PROGRAM PRG_METHOD
VAR
	(* Declarations for UA_Connect *)	
	fbUA_Connect: UA_Connect;
	SessionConnectInfo: ST_UASessionConnectInfo;
	nConnectionHdl: DWORD;
	
	(* Declarations for UA_GetNamespaceIndex *)
	fbUA_GetNamespaceIndex: UA_GetNamespaceIndex;
	nNamespaceIndex: UINT;
	
	(* Declarations for UA_MethodGetHandle *)
	fbUA_MethodGetHandle: UA_MethodGetHandle;
	ObjectNodeID: ST_UANodeID;
	MethodNodeID: ST_UANodeID;
	nMethodHdl: DWORD;
	
	(* Declarations for UA_MethodCall *)
	fbUA_MethodCall: UA_MethodCall;
	sObjectNodeIdIdentifier	: STRING(MAX_STRING_LENGTH) := 'MAIN.fbMathematics'; // change to object node identifier (UAObject above method)
	sMethodNodeIdIdentifier : STRING(MAX_STRING_LENGTH) := 'MAIN.fbMathematics#M_Mul'; // change to method node identifier (UAMethod to call)
	nAdrWriteData: PVOID;
	numberIn1: INT := 42; // change according to input value and data type
	numberIn2: INT := 42; // change according to input value and data type
	numberOutPro: DINT; // result (output parameter of M_Mul())
	cbWriteData: UDINT; // calculated automatically by M_Init()
	InputArguments: ARRAY[1..2] OF ST_UAMethodArgInfo; // change according to input parameters - M_Mul has 2 input parameters 
	stOutputArgInfo: ARRAY[1..1] OF ST_UAMethodArgInfo; // change according to output parameters - M_Mul has 1 output parameters
	stOutputArgInfoAndData: ST_OutputArgInfoAndData;
	nInputData: ARRAY[1..4] OF BYTE; // numberIn1(INT16)(2) + numberIn2(INT16)(2)
	nOffset: UDINT; // calculated by M_Init()
	nArg: INT; // used by M_Init()
	
	(* Declarations for UA_MethodReleaseHandle *)
	fbUA_MethodReleaseHandle: UA_MethodReleaseHandle;

	(* Declarations for UA_Disconnect *)
	fbUA_Disconnect: UA_Disconnect;
			
	(* Other Declarations *)
	bTest: BOOL := TRUE;
	bDone: BOOL;
	bBusy: BOOL;
	bError: BOOL;
	nErrorID: DWORD;
	iState: INT;
	RTrig: R_TRIG;
	bInputDataError: BOOL;
END_VAR
VAR CONSTANT
	nInputArgSize: INT := 4; // numberIn1(INT16)(2) + numberIn2(INT16)(2)
	nNumberOfInputArguments: DINT := 2; // change to number of input parameters - M_Mul has 2 input parameters
	nNumberOfOutputArguments: DINT := 1; // change to number of output parameters - M_Mul has 1 output parameters
END_VAR

CASE iState OF

0:	(* idle *)
	IF bTest THEN
		bTest		:= FALSE;
		bError		:= FALSE;
		nErrorID	:= 0;

		SessionConnectInfo.tConnectTimeout 		:= T#1M;
		SessionConnectInfo.tSessionTimeout 		:= T#1M;
		SessionConnectInfo.sApplicationName		:= '';
		SessionConnectInfo.eSecurityMode 		:= eUASecurityMsgMode_None;
		SessionConnectInfo.eSecurityPolicyUri 	:= eUASecurityPolicy_None;
		SessionConnectInfo.eTransportProfileUri := eUATransportProfileUri_UATcp;

		iState	:= iState + 1;
	END_IF

	
1:	(* open UA session *)
	fbUA_Connect(
		Execute				:= TRUE,
		ServerURL			:= sOpcUaServerUrl,
		SessionConnectInfo	:= SessionConnectInfo,
		Timeout				:= T#2M,
		ConnectionHdl		=> nConnectionHdl
	);

	IF NOT fbUA_Connect.Busy THEN
		fbUA_Connect(Execute := FALSE);

		IF NOT fbUA_Connect.Error THEN
			(* connected *)
			iState := iState + 1;
		ELSE
			bError			:= TRUE;
			nErrorID		:= fbUA_Connect.ErrorID;
			nConnectionHdl	:= 0;
			iState 			:= 0; (* idle *)
		END_IF
	END_IF


2:	(* GetNS Index *)
	fbUA_GetNamespaceIndex(
		Execute			:= TRUE,
		ConnectionHdl	:= nConnectionHdl,
		NamespaceUri	:= sNamespaceUri,
		NamespaceIndex	=> nNamespaceIndex
	);

	IF NOT fbUA_GetNamespaceIndex.Busy THEN
		fbUA_GetNamespaceIndex(Execute := FALSE);

		IF NOT fbUA_GetNamespaceIndex.Error THEN
			(* namespace index read successfully *)
			iState 		:= iState + 1;
		ELSE
			bError		:= TRUE;
			nErrorID	:= fbUA_GetNamespaceIndex.ErrorID;
			iState 		:= 7; (* disconnect *)
		END_IF
	END_IF

	
3:	(* Get Method Handle *)
	ObjectNodeID.eIdentifierType := eUAIdentifierType_String;
	ObjectNodeID.nNamespaceIndex := nNamespaceIndex;
	ObjectNodeID.sIdentifier	 := sObjectNodeIdIdentifier;

	MethodNodeID.eIdentifierType := eUAIdentifierType_String;
	MethodNodeID.nNamespaceIndex := nNamespaceIndex;
	MethodNodeID.sIdentifier	 := sMethodNodeIdIdentifier;

	M_Init();
	IF bInputDataError = FALSE THEN
		iState 	:= iState + 1;
	ELSE
		bBusy		:= FALSE;  
		bError 		:= TRUE;
		nErrorID 	:= 16#70A; //out of memory
	END_IF

	
4:	(* Method Get Handle *)
	fbUA_MethodGetHandle(
			Execute			:= TRUE,
			ConnectionHdl	:= nConnectionHdl,
			ObjectNodeID	:= ObjectNodeID,
			MethodNodeID 	:= MethodNodeID,
			MethodHdl		=> nMethodHdl
		);
	IF NOT fbUA_MethodGetHandle.Busy THEN
		fbUA_MethodGetHandle(Execute := FALSE);

		IF NOT fbUA_MethodGetHandle.Error THEN
			(*  *)
			iState := iState + 1; (* Call Method *)
		ELSE
			bError		:= TRUE;
			nErrorID	:= fbUA_MethodGetHandle.ErrorID;
			iState	 	:= 6; (* Release method Handle *)
		END_IF
	END_IF


5:	(* Method Call *)
	stOutputArgInfo[1].nLenData := SIZEOF(stOutputArgInfoAndData.pro);
	fbUA_MethodCall(
		Execute					:= TRUE,
		ConnectionHdl			:= nConnectionHdl,
		MethodHdl				:= nMethodHdl,
		nNumberOfInputArguments := nNumberOfInputArguments,	
		pInputArgInfo			:= ADR(InputArguments),
		cbInputArgInfo			:= SIZEOF(InputArguments),
		pInputArgData			:= ADR(nInputData),
		cbInputArgData			:= cbWriteData,
		pInputWriteData			:= 0,
		cbInputWriteData		:= 0,
		nNumberOfOutputArguments:= nNumberOfOutputArguments,
		pOutputArgInfo			:= ADR(stOutputArgInfo),
		cbOutputArgInfo			:= SIZEOF(stOutputArgInfo),
		pOutputArgInfoAndData	:= ADR(stOutputArgInfoAndData),
		cbOutputArgInfoAndData	:= SIZEOF(stOutputArgInfoAndData),		
	);
	IF NOT fbUA_MethodCall.Busy THEN
		fbUA_MethodCall(Execute := FALSE);
		IF NOT fbUA_MethodCall.Error THEN
			(* clear data and restart *)
			iState := iState + 1; (* Release handle *)
			numberOutPro := stOutputArgInfoAndData.pro;
		ELSE
			bError		:= TRUE;
			nErrorID	:= fbUA_MethodCall.ErrorID;
			iState		:= 6; (* Release method handle *)
		END_IF
	END_IF


6:	(* Release Method Handle *)
	fbUA_MethodReleaseHandle(
		Execute			:= TRUE,
		ConnectionHdl	:= nConnectionHdl,
		MethodHdl		:= nMethodHdl
	);

	IF NOT fbUA_MethodReleaseHandle.Busy THEN
		fbUA_MethodReleaseHandle(Execute := FALSE);
		bBusy := FALSE;
		IF NOT fbUA_MethodReleaseHandle.Error THEN
			(* session closed *)
			iState 	:= 7; (* Disconnect *)
		ELSE
			bError		:= TRUE;
			nErrorID	:= fbUA_MethodReleaseHandle.ErrorID;
			iState 		:= 7; (* Disconnect *)
		END_IF
	END_IF
	
	
7:	(* Disconnect *) 
	fbUA_Disconnect(
		Execute			:= TRUE,
		ConnectionHdl	:= nConnectionHdl
	);

	IF NOT fbUA_Disconnect.Busy THEN
		fbUA_Disconnect(Execute := FALSE);

		IF NOT fbUA_Disconnect.Error THEN
			(* disconnected *)
			iState 	:= 0; (* idle *)
			bDone 	:= TRUE;
			bBusy 	:= FALSE;
		ELSE
			bBusy 			:= FALSE;
			bError			:= TRUE;
			nErrorID		:= fbUA_Disconnect.ErrorID;
			iState 			:= 0; (* idle *)
			nConnectionHdl	:= 0;
		END_IF
	END_IF
END_CASE

ACTION M_Init:
bInputDataError := FALSE; 
nOffset := 0;
MEMSET(ADR(InputArguments),0,SIZEOF(InputArguments));
MEMSET(ADR(nInputData),0,SIZEOF(nInputData));

nArg := 1;
(*numberIn1*)			(********** Input parameter 1 **********)
InputArguments[nArg].DataType			:= eUAType_Int16;
InputArguments[nArg].ValueRank			:= -1; 							(* Scalar = -1 or Array *)
InputArguments[nArg].ArrayDimensions[1]	:= 0; 							(* Number of Dimension in case its an array *)
InputArguments[nArg].nLenData			:= SIZEOF(numberIn1);			(* Length if its a STRING *)
IF nOffset + SIZEOF(numberIn1) > nInputArgSize THEN 
	bInputDataError := TRUE;
	RETURN;
ELSE
	MEMCPY(ADR(nInputData)+nOffset,ADR(numberIn1),SIZEOF(numberIn1));				(* VALUE in BYTES FORM *)
	nOffset := nOffset + SIZEOF(numberIn1);
END_IF

nArg := nArg + 1;
(* numberIn2;*)			(********** Input parameter 2 **********)
InputArguments[nArg].DataType			:= eUAType_Int16;
InputArguments[nArg].ValueRank			:= -1; 							(* Scalar = -1 or Array *)
InputArguments[nArg].ArrayDimensions[1]	:= 0; 							(* Number of Dimension in case its an array *)
InputArguments[nArg].nLenData			:= SIZEOF(numberIn2);				(* Length if its a STRING *)
IF nOffset + SIZEOF(numberIn2) > nInputArgSize THEN 
	bInputDataError := TRUE;
	RETURN;
ELSE
	MEMCPY(ADR(nInputData)+nOffset,ADR(numberIn2),SIZEOF(numberIn2));			(* VALUE in BYTES FORM *)
	nOffset := nOffset + SIZEOF(numberIn2);
END_IF

cbWriteData := nOffset;
END_ACTION

END_PROGRAM
